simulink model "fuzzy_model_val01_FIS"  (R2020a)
settings: Solver=VariableStepAuto  StartTime=0.0  StopTime=tfin  RelTol=1e-3
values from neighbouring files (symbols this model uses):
  Ts = 5    [sisopres.m]
undefined symbols (not defined in the file or in its folder): magnitude
libraries: fuzblock x1

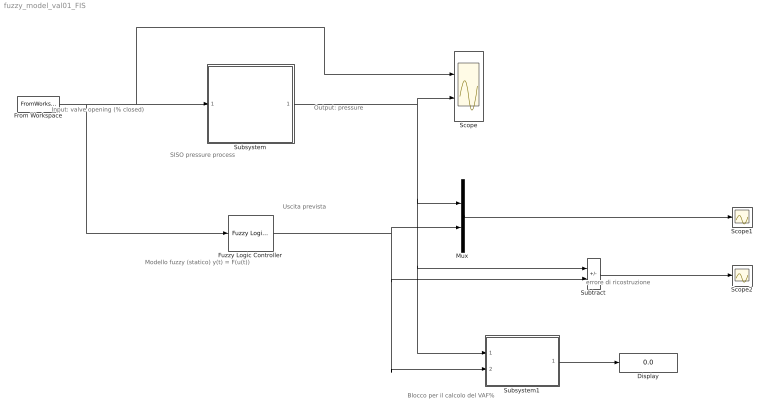
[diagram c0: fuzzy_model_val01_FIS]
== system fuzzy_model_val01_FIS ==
  note: Blocco per il calcolo del VAF%
  note: errore di ricostruzione
  note: Uscita prevista
  note: Modello fuzzy (statico) y(t) = F(u(t))
  note: Output: pressure
  note: Input: valve opening (% closed)
  note: SISO pressure process
  Display : Display
  From Workspace : FromWorkspace  VariableName=[tsim U]  SampleTime=Ts
  Fuzzy Logic Controller : fuzblock/Fuzzy Logic  Controller  FIS=FIS01  OutputSampleNumber=101  DataType=double  FuzzifiedInputs=off  RuleFiringStrengths=off  RuleOutputs=off  AggregatedOutputs=off  SimulateUsing=Interpreted execution  OutOfRangeInputValueMessage=warning  NoRuleFiredMessage=warning  EmptyOutputFuzzySetMessage=warning
  Mux : Mux  Inputs=2
  Scope : Scope  NumInputPorts=2
  Scope1 : Scope
  Scope2 : Scope
  Subsystem : Subsystem
  Subsystem1 : Subsystem
  Subtract : Sum  Inputs=+-
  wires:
  From Workspace/1 -> Fuzzy Logic Controller/1, Scope/1, Subsystem/1(u)
  Mux/1 -> Scope1/1
  Subtract/1 -> Scope2/1
  Fuzzy Logic Controller/1 -> Subsystem1/2(y_prev), Subtract/2, Mux/2
  Subsystem/1(y) -> Subsystem1/1(y_mis), Subtract/1, Mux/1, Scope/2
  Subsystem1/1(VAF%) -> Display/1

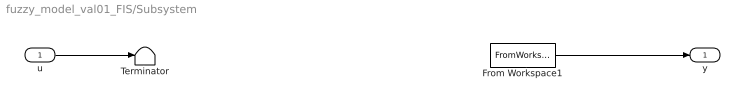
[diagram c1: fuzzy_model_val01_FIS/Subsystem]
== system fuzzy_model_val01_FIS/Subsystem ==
  u : Inport
  From Workspace1 : FromWorkspace  VariableName=[tsim Y]  SampleTime=Ts
  Terminator : Terminator
  y : Outport
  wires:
  From Workspace1/1 -> y/1
  u/1 -> Terminator/1

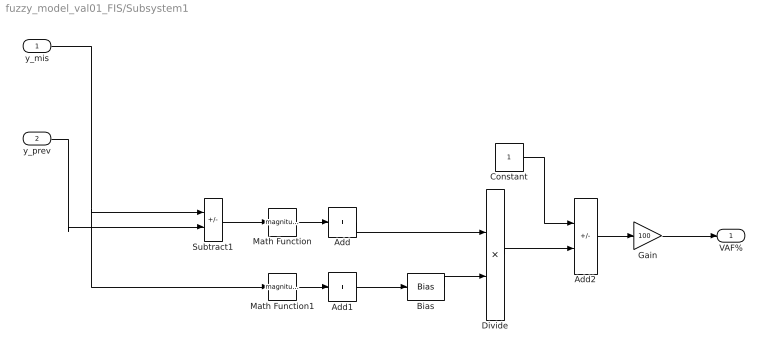
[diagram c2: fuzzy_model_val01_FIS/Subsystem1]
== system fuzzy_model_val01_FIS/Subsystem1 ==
  y_mis : Inport
  y_prev : Inport  Port=2
  Add : Sum  Inputs=+
  Add1 : Sum  Inputs=+
  Add2 : Sum  Inputs=+-
  Bias : Bias  Bias=1e-7
  Constant : Constant
  Divide : Product  Inputs=*/
  Gain : Gain  Gain=100
  Math Function : Math  Operator=magnitude^2
  Math Function1 : Math  Operator=magnitude^2
  Subtract1 : Sum  Inputs=+-
  VAF% : Outport
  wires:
  Add2/1 -> Gain/1
  Math Function/1 -> Add/1
  Bias/1 -> Divide/2
  y_mis/1 -> Math Function1/1, Subtract1/1
  Add1/1 -> Bias/1
  Math Function1/1 -> Add1/1
  Subtract1/1 -> Math Function/1
  Constant/1 -> Add2/1
  Divide/1 -> Add2/2
  Add/1 -> Divide/1
  y_prev/1 -> Subtract1/2
  Gain/1 -> VAF%/1
